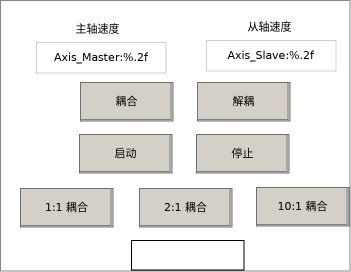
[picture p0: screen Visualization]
VISUALIZATION Visualization  // 351x272
    Label (58,14 79x30), "主轴速度"
    Textfield (36,42 130x31), "Axis_Master:%.2f", text variable: MAIN.Axis_Master.NcToPlc.ActVelo
    Label (230,12 79x30), "从轴速度"
    Textfield (206,40 130x31), "Axis_Slave:%.2f", text variable: MAIN.Axis_Slave.NcToPlc.ActVelo
    Button (79,134 93x39), "启动"
        tap MAIN.bStart
    Button (196,134 93x39), "停止"
        tap MAIN.bStop
    Button (20,188 93x39), "1:1 耦合"
        tap MAIN.bSwitch_1
    Button (139,188 93x39), "2:1 耦合"
        tap MAIN.bSwitch_2
    Button (256,187 93x39), "10:1 耦合"
        tap MAIN.bSwitch_3
    Button (80,82 93x39), "耦合"
        tap MAIN.bGearIn
    Button (197,82 93x39), "解耦"
        tap MAIN.bGearOut
    Rectangle (131,240 113x30), text list: 'Gear_Status', text index: MAIN.Axes_GearIn.InGear
END_VISUALIZATION
